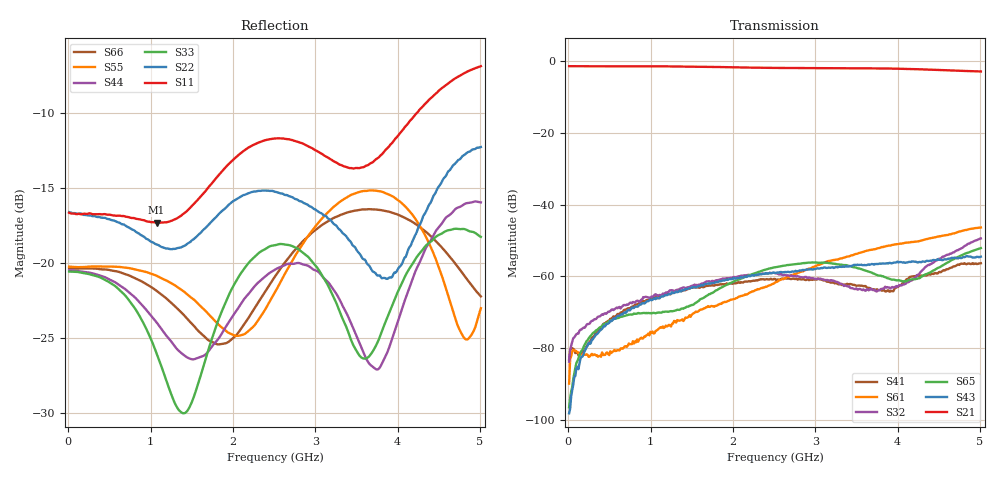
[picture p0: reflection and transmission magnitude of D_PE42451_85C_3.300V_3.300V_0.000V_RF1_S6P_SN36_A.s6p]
! Device ID: PE42451
! Serial: 36
! Insertion: A
! Temp: 85C
! VDD: 3.300
! Control_Hi: 100.000
! Control_Lo: 0.000
! Logic State: RF1
! Port 1: RFC
! Port 2: RF1
! Port 3: RF2
! Port 4: RF3
! Port 5: RF4
! Port 6: RF5
! V1 = 3.30
! V2 = 0.00
! V3 = 0.00
! V4 = 0.00
! IDD: 1.744150e-05
#  Hz  S  RI  R  50
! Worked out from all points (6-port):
!   401 points, 10 MHz to 5.01 GHz, reference 50 ohm
!   strongest paths, dB at 10 MHz, 1.26 GHz, 2.51 GHz, 3.76 GHz, 5.01 GHz:
!     S21: -1.5, -1.6, -2.0, -2.1, -3.0
!     S43: -98.1, -64.4, -59.0, -56.6, -54.5
!     S65: -96.4, -69.7, -57.5, -59.7, -52.1
!     S32: -83.7, -63.8, -59.1, -63.9, -49.4
!     S61: -89.8, -73.2, -61.7, -52.2, -46.4
!     S41: -83.2, -64.6, -60.7, -63.8, -56.3
!   lowest |S11| = -17.3 dB at 1.073 GHz (marker M1), VSWR 1.32, Z = 59.5 - j11.6 ohm
!   |S11| at or under -10 dB: start of sweep to 4.233 GHz
